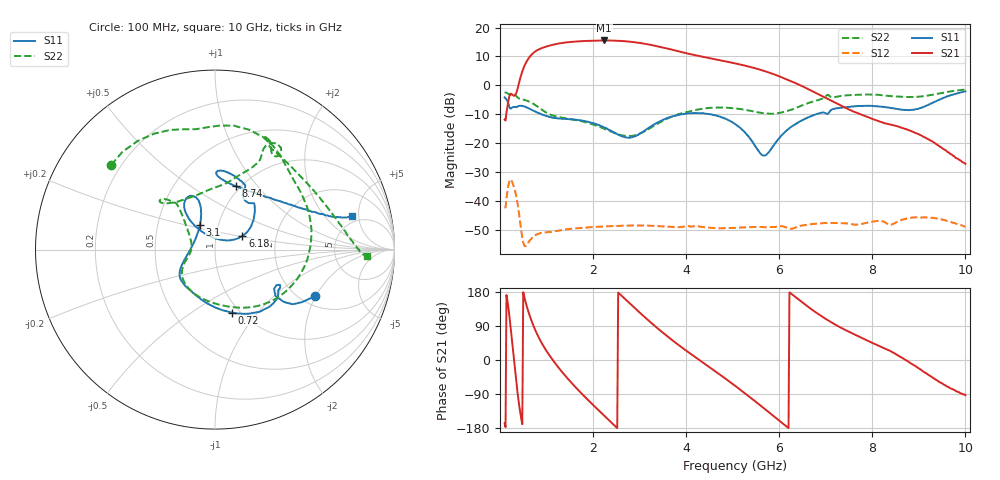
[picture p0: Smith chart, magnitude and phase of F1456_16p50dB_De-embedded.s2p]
! Integrated Device Technology
! Corporate Headquarters
! 6024 Silver Creek Valley Road
! San Jose, CA 95138  USA
! Phone:  1-408-284-8200
! Toll Free:  1-800-223-1366
! Webpage:  http://www.idt.com/
! Timing and RF Division
! 515 Groton Road, Suite 102
! Westford, MA 01886-6024
! Device:  F1456
! Description: 6-bit 0.5 dB Transmit Variable Gain Amplifier
! Frequency:  2100.0 -  2950.00 MHz
! Package:  6x6 mm Thin QFN Plastic Package: 28 pin
! State:  33
! Atten State:  16.5 dB
! Voltage:  +5.00 Volts
! Current:  216.972 mA
! Data:  The device was measured on a the F1455 evaluation board which has
!  individual transmission lines to the RF pins.  Data was collected
!  using a calibrated network analyzer.  The evaluation board was
!  de-embedded using a TRL calibration technique.
!  The reference plane is the edge of the package pin.
!  Pin  1 = CSb
!  Pin  2 = DATA
!  Pin  3 = CLK
!  Pin  4 = RSET
!  Pin  5 = GND
!  Pin  6 = RFIN  = Port 1
!  Pin  7 = GND
!  Pin  8 = NC
!  Pin  9 = NC
!  Pin 10 = NC
!  Pin 11 = NC
!  Pin 12 = NC
!  Pin 13 = NC
!  Pin 14 = /STBY
!  Pin 15 = GND
!  Pin 16 = RFOUT  = Port 2
!  Pin 17 = GND
!  Pin 18 = NC
!  Pin 19 = NC
!  Pin 20 = NC
!  Pin 21 = GND
!  Pin 22 = NC
!  Pin 23 = GND
!  Pin 24 = NC
!  Pin 25 = NC
!  Pin 26 = NC
!  Pin 27 = GND
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# GHz S dB R 50
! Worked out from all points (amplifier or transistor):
!   496 points, 100 MHz to 10 GHz, reference 50 ohm
!   highest |S21| = 15.5 dB at 2.24 GHz (marker M1)
!   |S21| within 3 dB of that: 846.4 MHz to 3.645 GHz (2.799 GHz wide, 125 % of centre)
!   unconditionally stable (mu >= 1): start of sweep to end of sweep
!   at 1.74 GHz: K = 22.63, MAG = 15.8 dB, |S12| = -49.4 dB
!   at 5.06 GHz: K = 49.59, MAG = 8.5 dB, |S12| = -49.4 dB
!   at 10 GHz: K = 356.91, MAG = -17.6 dB, |S12| = -49.0 dB
!   S11 on the Smith chart (normalised r, x): 100 MHz: 2.36, -1.98; 720 MHz: 0.92, -0.74; 3.1 GHz: 0.82, +0.23; 6.18 GHz: 1.34, +0.21; 8.74 GHz: 0.95, +0.78; 10 GHz: 4.22, +4.08
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0.1  -4.20 -25.0  -11.88 -166.9  -42.30 48.3  -2.55 140.8
0.32  -7.54 -31.6  -3.56 -18.6  -36.37 -148.9  -3.32 67.0
0.44  -7.09 -41.3  2.72 -142.1  -48.20 136.7  -4.73 38.1
0.56  -7.57 -56.9  7.86 148.7  -55.60 157.9  -5.21 11.7
0.72  -8.80 -75.2  11.23 90.2  -52.41 140.6  -6.45 -23.4
0.96  -10.47 -99.4  13.24 31.6  -51.04 96.0  -9.12 -67.6
1.18  -11.36 -116.6  14.21 -7.6  -50.60 71.3  -10.68 -95.5
1.48  -11.74 -133.1  14.96 -52.5  -49.82 46.8  -11.63 -123.2
1.76  -12.23 -143.8  15.30 -89.2  -49.40 28.9  -12.48 -139.9
2.24  -14.60 -159.6  15.54 -147.0  -48.94 3.5  -15.06 -158.7
2.64  -17.80 171.2  15.33 166.4  -48.67 -16.1  -17.41 -176.8
3.1  -15.82 121.2  14.42 114.3  -48.60 -38.6  -16.05 152.3
3.4  -12.80 109.8  13.46 82.3  -48.82 -52.9  -13.23 138.8
3.74  -10.64 108.7  12.16 48.6  -49.13 -67.1  -10.55 131.3
4.1  -9.68 114.0  10.75 16.2  -48.99 -82.9  -8.96 131.4
5.06  -13.51 130.5  7.57 -68.8  -49.38 -127.1  -8.01 138.9
5.66  -24.34 79.3  5.05 -126.3  -49.17 -161.1  -9.67 122.0
6.18  -15.39 26.4  1.88 -177.8  -49.52 166.3  -8.86 84.5
6.7  -10.61 41.9  -1.95 133.2  -48.13 142.2  -5.77 65.0
8.36  -7.76 87.8  -13.50 25.4  -48.30 70.8  -3.72 62.4
8.74  -8.56 71.9  -15.31 -1.8  -46.14 63.9  -4.05 49.0
10  -2.11 13.7  -27.23 -92.9  -49.03 -22.5  -1.46 -2.6
